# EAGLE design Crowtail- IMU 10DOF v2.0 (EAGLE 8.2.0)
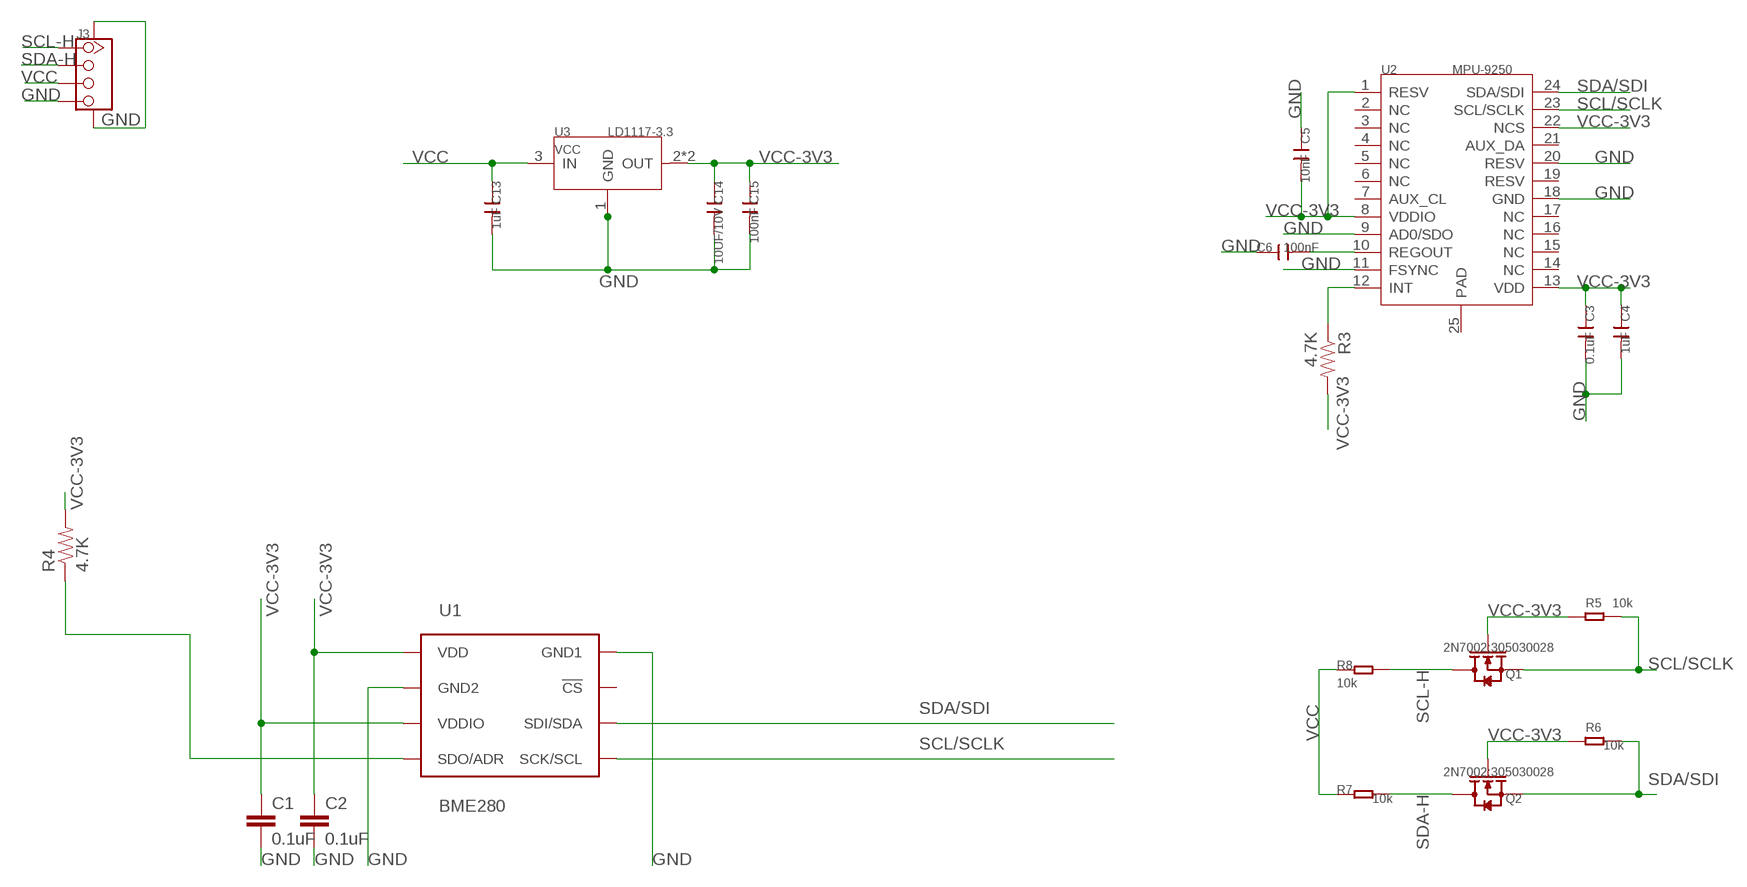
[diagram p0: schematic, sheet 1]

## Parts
C1  0.1uF  0.1UF-25V-5%(0603)  [0603-CAP]
C2  0.1uF  0.1UF-25V-5%(0603)  [0603-CAP]
C3  0.1uF  C-0603  [C0603]
C4  1uF  C-0603  [C0603]
C5  10nF  C-0603  [C0603]
C6  100nF  C-0603  [C0603]
C13  1uF  C-0603  [C0603]
C14  10UF/10V  C-0805  [C0805]
C15  100nF  C-0603  [C0603]
J3  TWIG-4P-2.0-SMD-FEMALE-REINFORCE'90D'  [4P-SMD-2.0-90D]
Q1  2N7002;305030028  MOSFET-N'SOT23'  [SOT-23]
Q2  2N7002;305030028  MOSFET-N'SOT23'  [SOT-23]
R3  4.7K  4.7KOHM-1/10W-1%(0603)  [0603-RES]
R4  4.7K  4.7KOHM-1/10W-1%(0603)  [0603-RES]
R5  10k  RES-0603  [R0603]
R6  10k  RES-0603  [R0603]
R7  10k  RES-0603  [R0603]
R8  10k  RES-0603  [R0603]
U1  BME280  [BME280_LGA]
U2  MPU-9250  [LEAD-QFN24]
U3  LD1117-3.3  LD1117'SOT89'  [SOT89]

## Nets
GND: C1.2 C2.2 C3.2 C4.2 C5.1 C6.1 C13.2 C14.2 C15.2 J3.4 J3.SS1 J3.SS2 U1.P$1(GND1) U1.P$7(GND2) U2.9(AD0/SDO) U2.11(FSYNC) U2.18(GND) U2.20(RESV) U3.1(GND)
N$1: C6.2 U2.10(REGOUT)
N$2: R3.1 U2.12(INT)
SCL-H: J3.1 Q1.3(D) R8.2
SCL/SCLK: Q1.2(S) R5.2 U1.P$4(SCK/SCL) U2.23(SCL/SCLK)
SDA-H: J3.2 Q2.3(D) R7.2
SDA/SDI: Q2.2(S) R6.2 U1.P$3(SDI/SDA) U2.24(SDA/SDI)
SDO/ADR: R4.1 U1.P$5(SDO/ADR)
VCC: C13.1 J3.3 R7.1 R8.1 U3.3(IN)
VCC-3V3: C1.1 C2.1 C3.1 C4.1 C5.2 C14.1 C15.1 Q1.1(G) Q2.1(G) R3.2 R4.2 R5.1 R6.1 U1.P$6(VDDIO) U1.P$8(VDD) U2.1(RESV) U2.8(VDDIO) U2.13(VDD) U2.22(NCS) U3.2(OUT) U3.4(OUT)
Unconnected: U1.P$2(!CS) U2.2(NC) U2.3(NC) U2.4(NC) U2.5(NC) U2.6(NC) U2.7(AUX_CL) U2.14(NC) U2.15(NC) U2.16(NC) U2.17(NC) U2.19(RESV) U2.21(AUX_DA) U2.25(PAD)

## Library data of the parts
C1 C2 = SparkFun-Capacitors:0.1UF-25V-5%(0603): CAP-08604; PROD_ID: CAP-08604
C3-C6 C13-C15 = Discrete:C*: Ceramic Capacitors
J3 = Connector:TWIG-4P-2.0-SMD-FEMALE-REINFORCE
Q1 Q2 = Discrete-new:MOSFET-N: IRLL014: http://www.vishay.com/docs/91319/sihll014.pdf
R3 R4 = SparkFun-Resistors:4.7KOHM-1/10W-1%(0603): RES-07857; PROD_ID: RES-07857
R5-R8 = Discrete-new:RES
U1 = BME280ComponentLibrary:BME280; PROD_ID: IC-13090
U2 = template:MPU-9250
U3 = IC:LD1117: Low Drop Fixed And Adjustable Positive Voltage Regulators http://www.datasheetcatalog.org/datasheet/SGSThomsonMicroelectronics/mXuqtqv.pdf

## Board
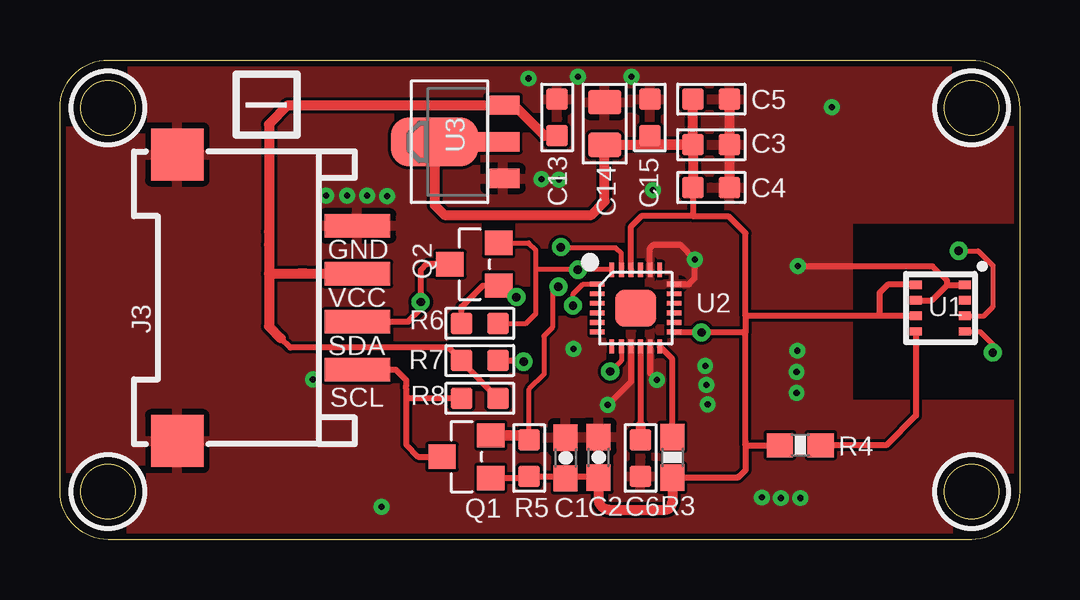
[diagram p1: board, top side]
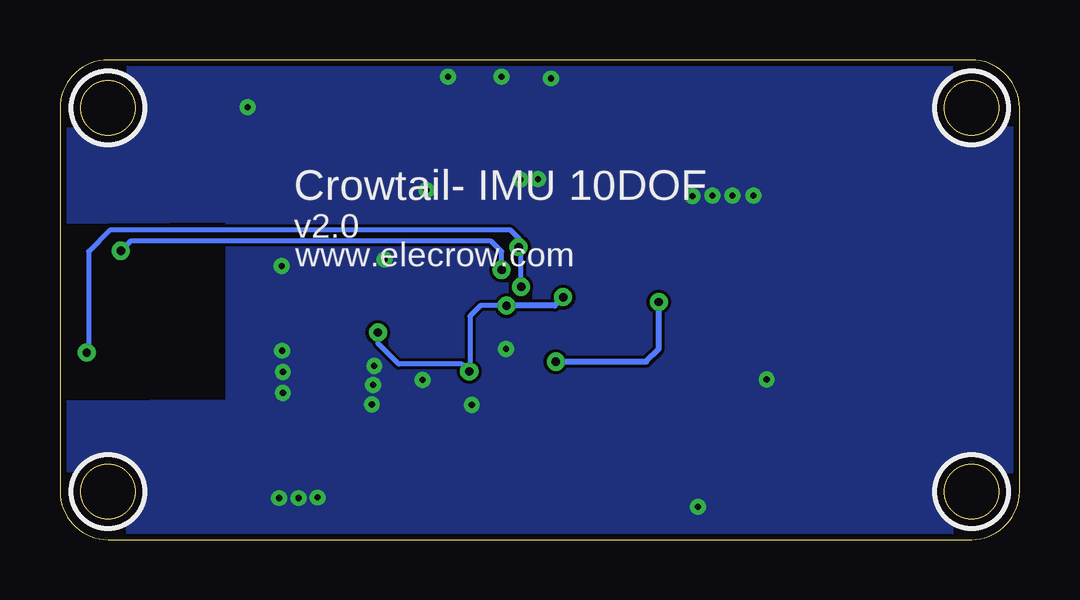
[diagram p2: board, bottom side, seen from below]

Size 40 x 20 mm. Coordinates in mm from the lower left corner, seen from the top.
Outline: 2,20 38,20 arc-90 40,18 40,2 arc-90 38,0 2,0 arc-90 0,2 0,18 arc-90 2,20
Outline: circle at 38,18 radius 1.14
Outline: circle at 38,2 radius 1.14
Outline: circle at 2,18 radius 1.14
Outline: circle at 2,2 radius 1.14
Copper layers (1*16): Top 0.035mm / dielectric 1.5mm / Bottom 0.035mm
Design rules "default": minimum track width 10mil, minimum drill 10mil, track to track 5mil, track to pad 5mil, pad to pad 5mil, via to via 5mil, smd to smd 0mil, copper to edge 10mil, drill to drill 8mil, minimum pad ring 10mil, minimum via ring 8mil, stop-mask expansion 4mil, vias tented up to drill 100mil, thermal gap 10mil
tRestrict: area 36.5,16.5 to 39.5,19.5; area 36.5,0.5 to 39.5,3.5; area 0.5,16.5 to 3.5,19.5; area 0.5,0.5 to 3.5,3.5
bRestrict: area 36.5,16.5 to 39.5,19.5; area 36.5,0.5 to 39.5,3.5; area 0.5,16.5 to 3.5,19.5; area 0.5,0.5 to 3.5,3.5

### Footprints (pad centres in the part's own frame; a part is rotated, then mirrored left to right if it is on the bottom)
0603-CAP = smd 1.1 x 1: 1 -0.85,0; 2 0.85,0
C0603 = smd 0.889 x 0.889: 1 -0.762,0; 2 0.762,0
C0805 = smd 1.016 x 1.397: 1 -0.889,0; 2 0.889,0
4P-SMD-2.0-90D = smd 0.965 x 2.74: 1 -3,-0.1; 2 -1,-0.1; 3 1,-0.1; 4 3,-0.1 | smd 2.159 x 2.184: SS1 -5.974,7.4; SS2 5.974,7.4
SOT-23 = smd 1.016 x 1.143: 1 -0.889,-1.016; 2 0.889,-1.016; 3 0,1.016
0603-RES = smd 1.1 x 1: 1 -0.85,0; 2 0.85,0
R0603 = smd 0.889 x 0.889: 1 0,0.762; 2 0,-0.762
BME280_LGA = smd 0.5 x 0.35: P$1 1.025,0.975; P$2 1.025,0.325; P$3 1.025,-0.325; P$4 1.025,-0.975; P$5 -1.025,-0.975; P$6 -1.025,-0.325; P$7 -1.025,0.325; P$8 -1.025,0.975
LEAD-QFN24 = smd 0.6 x 0.2: 1 -1.6,1; 2 -1.6,0.6; 3 -1.6,0.2; 4 -1.6,-0.2; 5 -1.6,-0.6; 6 -1.6,-1; 13 1.6,-1; 14 1.6,-0.6; 15 1.6,-0.2; 16 1.6,0.2; 17 1.6,0.6; 18 1.6,1 | smd 0.2 x 0.6: 7 -1,-1.6; 8 -0.6,-1.6; 9 -0.2,-1.6; 10 0.2,-1.6; 11 0.6,-1.6; 12 1,-1.6; 19 1,1.6; 20 0.6,1.6; 21 0.2,1.6; 22 -0.2,1.6; 23 -0.6,1.6; 24 -1,1.6 | smd 1.7 x 1.54: 25 0,0
SOT89 = smd 0.8 x 1.4: 1 -1.524,-1.905; 3 1.524,-1.905 | smd 0.8 x 1.9: 2 0,-1.651 | smd 2.032 x 3.65: 4 0,0.94

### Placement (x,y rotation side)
C1  21.08,3.4 90 top
C2  22.45,3.43 90 top
C3  27.15,16.46 0 top
C4  27.15,14.68 0 top
C5  27.15,18.36 180 top
C6  24.21,3.4 90 top
C13  20.73,17.6 90 top
C14  22.71,17.35 90 top
C15  24.59,17.6 90 top
J3  12.29,10.08 90 top
Q1  16.94,3.45 90 top
Q2  17.27,11.48 90 top
R3  25.53,3.43 270 top
R4  30.86,3.94 180 top
R5  19.56,3.4 180 top
R6  17.5,9.02 90 top
R7  17.5,7.47 90 top
R8  17.5,5.89 270 top
U1  36.7,9.65 0 top
U2  24,9.65 0 top
U3  16.56,16.59 90 top

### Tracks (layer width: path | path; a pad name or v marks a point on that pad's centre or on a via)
GND  (via drill 0.25)
  Top 0.254: U2.9 23.8,6.58 v22.84,5.61 | U2.11 24.6,6.94 v24.89,6.66 | U2.20 24.6,12.16 24.74,12.29 25.86,12.29 v26.47,11.68 26.47,10.9 26.22,10.65 U2.18 | U1.P$7 36.34,9.98 36.98,10.62 | 36.98,10.62 37.72,10.62 U1.P$1 | v30.76,11.4 36.37,11.4 36.98,10.79 36.98,10.62
  Top 0.406: C5.1 C3.2 C4.2
  other vias: 13.41,1.37 32.18,18.03 10.54,6.68 29.26,1.75 30.05,1.73 30.86,1.73 26.9,7.24 26.95,6.45 27,5.64 30.73,7.87 30.71,6.99 30.71,6.12 21.41,7.95 24.71,14.58 20.07,15.04 20.8,15.01 19.53,19.23 21.59,19.3 23.83,19.3 11.1,14.35 11.96,14.35 12.8,14.35 13.64,14.33
  pour Bottom: 39.57,5.61 32.89,5.66 32.89,13.41 40.54,13.34 40.77,13.34 40.77,17.83 arc90 38.02,20.57 2.24,20.57 2.24,20.6 arc90 -0.61,17.75 -0.61,17.58 -0.64,17.58 -0.64,2.06 arc90 2.16,-0.74 37.8,-0.74 37.8,-0.79 arc90 40.67,2.08 40.67,5.66
  pour Top: 32.87,13.39 40.77,13.39 40.77,18.29 arc90 38.56,20.5 2.11,20.5 arc90 -0.51,17.88 -0.51,1.88 arc90 2.08,-0.71 38.1,-0.71 arc90 40.61,1.8 40.61,5.61 32.87,5.61
N$1
  Top 0.254: U2.10 24.2,4.78 | 24.2,4.12 24.21,4.12
  Top 0.406: 24.2,4.78 24.2,4.12 arc90 24.21,4.12 C6.2
N$2
  Top 0.254: R3.1 25.53,7.53 U2.12
SCL-H
  Top 0.254: 14.43,5.94 14.43,5.41 | 14.43,6.27 14.43,6.43 | 14.43,6.27 14.43,5.94 | R8.2 14.48,5.89 14.43,5.94 | 14.43,6.27 14.43,5.41 | 14.43,6.27 14.43,6.43 | 14.43,6.43 14.43,6.66 14,7.08 J3.1 | Q1.3 14.94,3.45 14.43,3.96 14.43,5.41
SCL/SCLK  (via drill 0.35)
  Top 0.203: U2.23 23.4,11.93 23.16,12.17 20.88,12.17 20.85,12.19 v20.88,12.19 | R5.2 19.56,4.34 19.56,6.27 20.17,6.88 20.17,8.48 20.55,8.87 20.55,10.31 v20.78,10.54 | U1.P$4 38.35,8.68 38.89,8.14 v38.89,7.8
  Top 0.406: R5.2 arc45 19.13,4.34 Q1.2 19.56,4.34
  Bottom 0.203: v20.78,10.54 20.78,12.09 v20.88,12.19 20.88,12.57 21.21,12.9 37.92,12.9 38.81,12.01 38.81,7.87 v38.89,7.8
SDA-H  (via drill 0.35)
  Top 0.254: J3.2 14.52,9.08 15.04,9.6 v15.04,9.91 15.04,11.23 15.29,11.48 Q2.3 | R7.2 19.3,7.47 19.33,7.44 v19.33,7.42
  Bottom 0.254: v19.33,7.42 16.82,7.42 15.57,7.42 15.04,7.95 v15.04,9.91
SDA/SDI  (via drill 0.35)
  Top 0.203: Q2.2 19.53,12.37 19.84,12.06 19.84,11.3 | 19.84,11.3 19.84,9.42 19.43,9.02 R6.2 | U2.24 v21.59,11.25 19.89,11.25 19.84,11.3 | v37.47,12.04 38.28,12.04 38.89,11.43 38.89,9.7 38.51,9.32 38.5,9.33 U1.P$3
  Bottom 0.203: v21.59,11.25 21.59,12.01 22.02,12.45 37.06,12.45 v37.47,12.04
SDO/ADR
  Top 0.254: U1.P$5 35.68,5.17 34.44,3.94 R4.1
VCC
  Top 0.254: R8.1 16.74,7.42 R7.1 16.2,8 9.6,8 9.21,8.39 | 8.71,8.89 8.71,11.07 8.71,12.29
  Top 0.406: 9.92,11.08 10.29,11.08 J3.3 8.71,11.07 | 8.71,12.83 8.71,17.32 9.5,18.11 U3.3 18.92,18.11 20.19,16.84 C13.1 | 8.71,12.83 8.71,12.29 | 8.71,12.83 8.71,8.89 9.21,8.39
VCC-3V3  (via drill 0.35)
  Top 0.203: U2.8 23.4,7.45 22.91,6.96 22.91,6.99 v22.94,7.01 | U2.1 21.8,10.65 21.39,10.24 v21.39,9.75
  Top 0.254: U1.P$6 34.16,9.33 | 34.16,9.33 28.57,9.33 | 28.57,8.64 v26.75,8.64 25.62,8.64 U2.13 28.56,8.65 28.57,8.64 | U1.P$8 34.5,10.63 34.16,10.29 34.16,9.33 | 28.57,3.94 28.57,4.09 28.57,8.64 | 28.57,9.33 28.57,8.64 | 28.57,3.94 R4.2 | Q1.1 19.48,2.56 R5.1 20.99,2.64 | 20.99,2.64 C1.1 | 20.99,2.64 22.39,2.64 C2.1 | C14.1 23.01,16.51 23.04,16.54 22.86,16.54 | R6.1 16.74,9.7 17.63,10.59 Q2.1 18.77,10.11 v19.02,10.11 | 28.57,9.33 28.57,12.78 27.86,13.49 26.39,13.49 | 26.39,13.49 24.23,13.49 23.8,13.06 U2.22 | C4.1 26.39,13.49 | R3.2 28.26,2.58 28.32,2.64 28.57,2.9 28.57,3.94
  Top 0.406: U3.2 U3.4 15.62,13.95 16.03,13.54 22.15,13.54 22.71,14.1 C14.1 24.21,16.46 | C3.1 C5.2 | C3.1 C4.1 | 24.21,16.46 C15.1 24.97,16.46 C3.1 | 24.21,16.46 C3.1 | C2.1 22.45,1.68 arc90 22.89,1.25 25.22,1.25 arc90 25.5,1.52 arc90 25.53,1.55 R3.2
  Bottom 0.203: v26.75,8.64 26.75,8.18 25.88,7.32 23.24,7.32 v22.94,7.01 22.91,7.04 22.91,9.32 22.48,9.75 v21.39,9.75
  Bottom 0.254: v19.02,10.11 19.38,9.75 v21.39,9.75

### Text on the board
tPlace: I | GND | VCC | SDA | SCL
bNames: Crowtail- IMU 10DOF | v2.0 | www.elecrow.com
